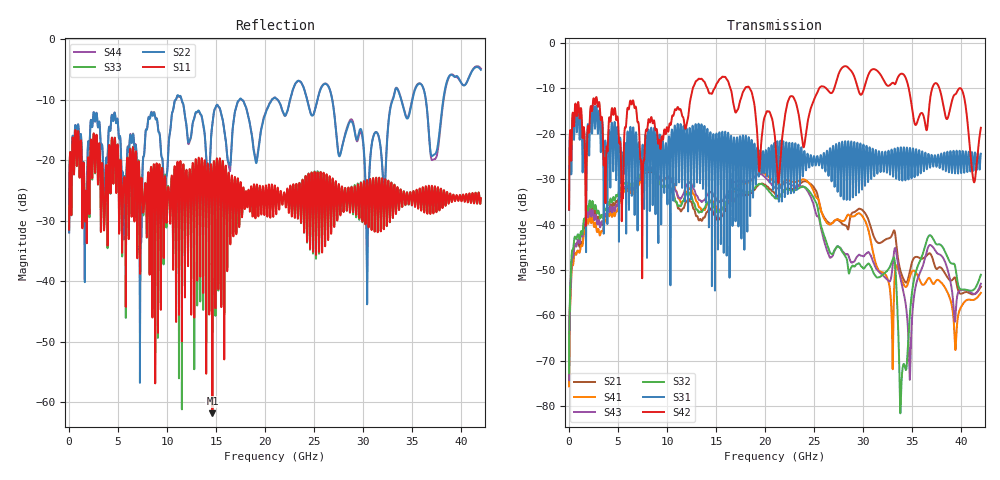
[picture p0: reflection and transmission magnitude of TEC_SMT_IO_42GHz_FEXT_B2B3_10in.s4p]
!! CHANNEL DESCRIPTION: Next Generation 28Gbps High Density SMT I/O Connector
!!  with 10" 5-6-5 Megatron 6 Stripline trace on host side and 1.25" 7-5-7 Megtron 6 Microstrip trace on plug side at 14GHz
!! HOST PCB DESCRIPTION: PCB thickness 2.86 mm, Nelco 4000-13SI (Dk 3.32, Df 0.010)
!!  23 Layer Board, 12 GND planes, 2 Layer route-out on Layers 10,12, 8 mil stub on vias
!!  Pairs on following layers
!!  Layer 10 - B2B3
!! CONNECTOR DESCRIPTION:  Next Generation 28Gbps High Density SMT I/O Connector
!! PLUG-IN CARD DESCRIPTION:  PCB thickness 1mm thick, Nelco 4000-13SI (Dk 3.32, Df 0.010)
!!  6 Layer Board, 4 GND planes, 0.35 x 1.4mm mating pads
!!  Micro-strip diff traces referenced to GND plane 3mils down, 2nd GND plane 15mils from top of board
!!  PCB GND planes are symmetric
!! MODEL DESCRIPTION: TE Connectivity S-parameter model produced from Macro-model
!! MODEL DATE: 9/25/2014 CR1a_GC1i, VR6&12_4
!! MODEL STATUS: Developmental
!! MODEL GEOMETRY: 2 Rows - Rows A, B. 3 pairs in each row, 6 total pairs
!! MODEL FREQUENCY RANGE: DC to 42 GHz in 10 MHz frequency steps
!! MODEL EDGE RATE LIMITATION: 11.90 ps (Using conservative 0.5/Fmax rule of thumb)
!! TIME-DOMAIN TRANSFORM CAUTIONS:
!! 1.) Do not simulate transient edge rates faster than the number listed above.  Edge
!!  rates faster than this number contain significant spectral content at frequencies
!!  above the model's highest frequency.
!! 2.) Even when simulating edge rates that are slower than the number listed above, be
!!  aware that the best time resolution possible with a direct iFFT is (1 / 2Fmax).
!!  As a result, time resolution is typically not adequate for most time-domain
!!  simulations unless tricks such as frequency-domain zero-padding and windowing are
!!  used to minimize leakage and aliasing.
!! 3.) Because the model has a uniform frequency step, a direct iFFT will result in an
!!  impulse that that has a time length given by either (1 / Fstep) or (1 / 2Fstep),
!!  depending on the transform being used.  Care has been taken in selecting the
!!  frequency step to ensure a settled impulse response for the model.  Therefore,
!!  convolution with the model's impulse response should present no issues.  However,
!!  if directly concatenating s-parameter models in the frequency domain a user must
!!  either interpolate necessary interim frequencies or complete impulse response
!!  zero-padding.  Impulse response zero-padding is more difficult, but more accurate.
!! PORT DEFINITIONS:
!! Port  1  ----->  Host, Bot Row  B2  B5  Module, Top Row  <-----  Port  2
!! Port  3  ----->  Host, Bot Row  B3  B6  Module, Top Row  <-----  Port  4
# Hz S MA R 50
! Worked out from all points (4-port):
!   4200 points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, 10 MHz to 42 GHz, reference 50 ohm
!   strongest paths, dB at 10 MHz, 10.51 GHz, 21.01 GHz, 31.51 GHz, 42 GHz:
!     S42: -36.7, -16.2, -21.0, -6.3, -18.7
!     S31: -36.8, -19.2, -23.7, -26.4, -24.4
!     S32: -72.7, -33.0, -34.2, -51.6, -51.0
!     S43: -74.2, -30.7, -32.0, -50.2, -53.0
!     S41: -75.6, -30.6, -30.8, -49.8, -55.0
!     S21: -74.0, -33.0, -33.3, -44.0, -53.7
!   lowest |S11| = -61.9 dB at 14.62 GHz (marker M1), VSWR 1.00, Z = 50.1 + j0.00489 ohm
!   |S11| at or under -10 dB: start of sweep to end of sweep
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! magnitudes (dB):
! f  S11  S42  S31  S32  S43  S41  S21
! 10 MHz  -31.5  -36.7  -36.8  -72.7  -74.2  -75.6  -74.0
! 2.22 GHz  -16.6  -14.0  -15.0  -36.1  -37.7  -39.4  -37.3
! 14.62 GHz  -61.9  -11.0  -26.5  -35.3  -33.0  -34.7  -36.8
! 33.06 GHz  -28.4  -8.8  -29.4  -47.3  -47.8  -63.7  -41.6
! 33.89 GHz  -26.0  -6.8  -24.2  -75.5  -52.8  -52.0  -50.8
! 36.67 GHz  -24.4  -15.5  -24.5  -42.6  -44.8  -51.8  -46.4
! 42 GHz  -26.3  -18.7  -24.4  -51.0  -53.0  -55.0  -53.7
